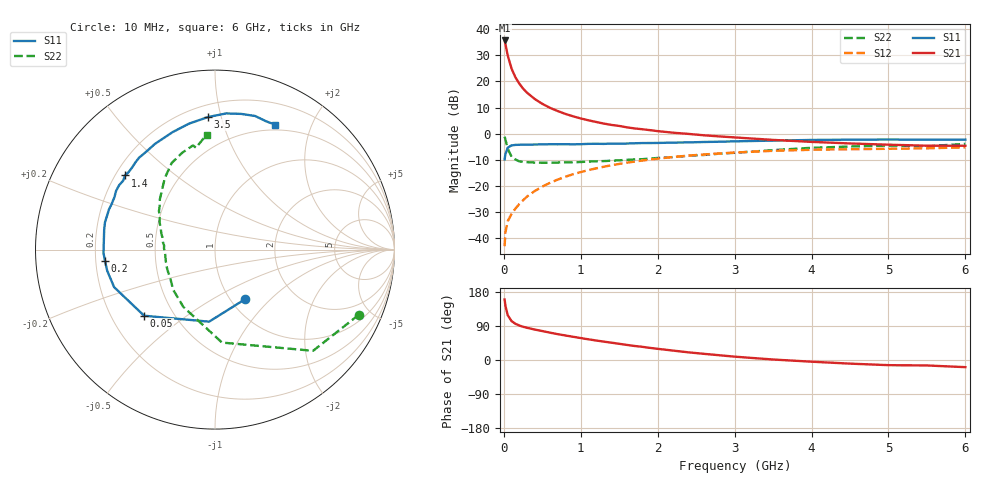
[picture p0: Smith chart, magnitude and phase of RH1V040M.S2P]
! SIEMENS Small Signal Semiconductors
! BFR106
! Si NPN RF Bipolar Junction Transistor in SOT23
! VCE = 1 V  IC = 40 mA
! Common Emitter S-Parameters:  August  1996
# GHz  S  MA  R  50
!  f  S11  S21  S12  S22
! GHz  MAG  ANG  MAG  ANG  MAG  ANG  MAG  ANG
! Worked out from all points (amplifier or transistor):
!   36 points, 10 MHz to 6 GHz, reference 50 ohm
!   highest |S21| = 35.7 dB at 10 MHz (marker M1)
!   |S21| within 3 dB of that: start of sweep to 31.72 MHz
!   unconditionally stable (mu >= 1): 231.8 MHz to end of sweep
!   at 250 MHz: K = 1.02, MAG = 20.5 dB, |S12| = -25.4 dB
!   at 1.4 GHz: K = 1.08, MAG = 6.0 dB, |S12| = -12.0 dB
!   at 6 GHz: K = 1.02, MAG = -0.6 dB, |S12| = -5.2 dB
!   S11 on the Smith chart (normalised r, x): 10 MHz: 1.16, -0.72; 50 MHz: 0.34, -0.35; 200 MHz: 0.24, -0.05; 1.4 GHz: 0.24, +0.34; 3.5 GHz: 0.28, +0.91; 6 GHz: 0.43, +1.50
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0.01  0.3232 -58.9  60.74 159.6  0.0071 75.2  0.8795 -24.4
0.02  0.4029 -94.7  52.41 144.0  0.013 64.6  0.7852 -45.9
0.05  0.5401 -137.0  31.58 118.3  0.0212 52.2  0.5194 -85.7
0.1  0.5998 -159.6  17.64 102.7  0.0294 55.3  0.3646 -119.0
0.15  0.612 -168.9  12.02 95.6  0.037 58.4  0.3228 -136.3
0.2  0.6158 -174.0  9.135 91.1  0.0452 62.3  0.2974 -146.5
0.25  0.6216 -178.2  7.305 87.7  0.0535 64.4  0.2895 -154.6
0.3  0.6204 179.0  6.126 85.1  0.0627 66.3  0.2863 -159.3
0.4  0.6224 173.8  4.637 80.4  0.08 67.6  0.2816 -166.8
0.5  0.6271 170.0  3.731 76.4  0.0977 67.7  0.279 -172.0
0.6  0.6316 166.0  3.132 72.1  0.1152 67.2  0.279 -175.5
0.7  0.6303 162.4  2.717 68.2  0.133 66.2  0.282 -178.5
0.9  0.6292 156.1  2.154 61.3  0.1683 63.6  0.2843 175.4
1.1  0.6409 149.3  1.807 54.5  0.2017 60.5  0.2939 171.5
1.4  0.6492 140.5  1.474 45.7  0.25 55.3  0.3057 165.3
1.7  0.6581 132.3  1.265 37.0  0.2937 50.1  0.3228 159.2
2.2  0.6774 119.6  1.048 24.8  0.3595 41.0  0.3576 149.5
2.8  0.7039 105.9  0.89 12.6  0.42 30.6  0.416 137.6
3.5  0.7396 93.0  0.763 1.3  0.472 19.6  0.4866 125.1
4.5  0.7701 79.0  0.653 -9.6  0.5063 5.8  0.5697 108.7
5.5  0.7695 68.1  0.591 -14.4  0.5273 -2.3  0.5773 100.6
6  0.7727 64.3  0.589 -18.9  0.5495 -8.8  0.6417 94.2
